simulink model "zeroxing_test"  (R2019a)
settings: Solver=VariableStepDiscrete  StartTime=0.0  StopTime=10  FixedStep=0.02  RelTol=1e-3  AbsTol=1e-6
StartFcn:
  | set_param('zeroxing_test/Scope','Open','on')

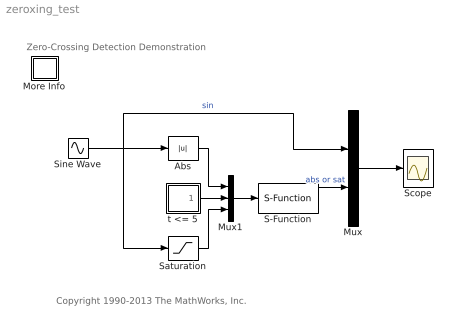
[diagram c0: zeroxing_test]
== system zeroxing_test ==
  note: Zero-Crossing Detection Demonstration
  note: Copyright 1990-2013 The MathWorks, Inc.
  Abs : Abs
  More Info : Subsystem
  Mux : Mux  Inputs=2
  Mux1 : Mux  Inputs=3
  S-Function : S-Function  FunctionName=zeroxingCtrl  SFunctionDeploymentMode=off  EnableBusSupport=off
  Saturation : Saturate  UpperLimit=[0.5 .55 .6]  LowerLimit=[-0.5 -.55 -.6]
  Scope : Scope
  Sine Wave : Sin  Phase=[.1 .2 .3]  SampleTime=0
  t <= 5 : Subsystem
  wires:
  t <= 5/1(t <= 5) -> Mux1/2
  S-Function/1 -> Mux/2  "abs or sat"
  Saturation/1 -> Mux1/3
  Abs/1 -> Mux1/1
  Sine Wave/1 -> Abs/1, Mux/1, Saturation/1  "sin"
  Mux/1 -> Scope/1
  Mux1/1 -> S-Function/1

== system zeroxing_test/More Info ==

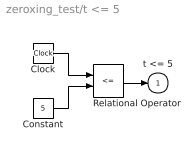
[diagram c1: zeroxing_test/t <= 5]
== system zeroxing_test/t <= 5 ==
  Clock : Clock
  Constant : Constant  Value=5
  Relational Operator : RelationalOperator  Operator=<=
  t <= 5 : Outport  InitialOutput=0
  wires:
  Constant/1 -> Relational Operator/2
  Clock/1 -> Relational Operator/1
  Relational Operator/1 -> t <= 5/1
